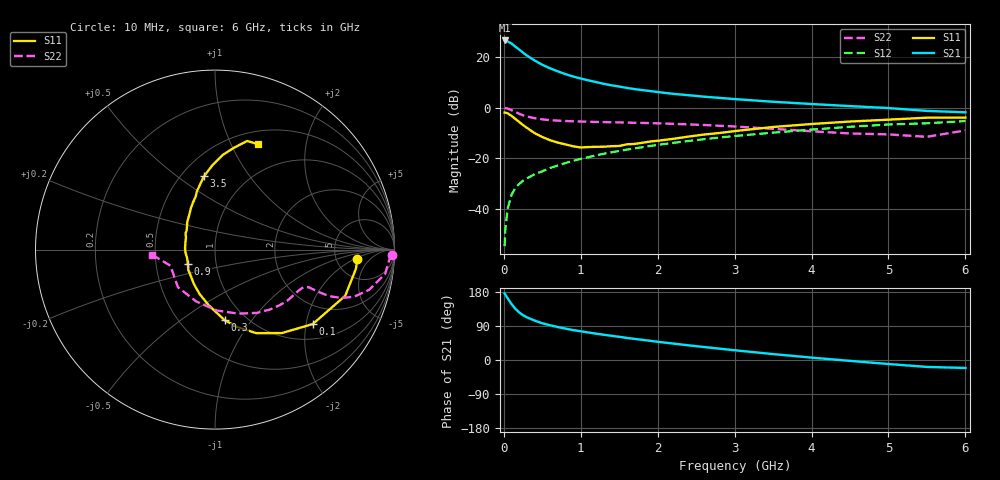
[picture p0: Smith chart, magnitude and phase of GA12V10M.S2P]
! Infineon Technologies  Discrete & RF Semiconductors
! BF775
! Si NPN RF Bipolar Junction Transistor in SOT23
! VCE = 12 V  IC = 10 mA
! Common Emitter S-Parameters:  May  1996
# GHz  S  MA  R  50
!  f  S11  S21  S12  S22
! GHz  MAG  ANG  MAG  ANG  MAG  ANG  MAG  ANG
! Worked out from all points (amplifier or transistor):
!   36 points, 10 MHz to 6 GHz, reference 50 ohm
!   highest |S21| = 26.6 dB at 10 MHz (marker M1)
!   |S21| within 3 dB of that: start of sweep to 173.5 MHz
!   unconditionally stable (mu >= 1): 658.7 MHz to 2.732 GHz
!   at 250 MHz: K = 0.64, MSG = 25.3 dB, |S12| = -28.9 dB
!   at 1.4 GHz: K = 1.09, MAG = 11.4 dB, |S12| = -17.7 dB
!   at 6 GHz: K = 0.87, MSG = 1.7 dB, |S12| = -5.3 dB
!   S11 on the Smith chart (normalised r, x): 10 MHz: 8.07, -2.38; 100 MHz: 1.40, -2.19; 300 MHz: 0.80, -0.75; 900 MHz: 0.73, -0.12; 3.5 GHz: 0.64, +0.63; 6 GHz: 0.65, +1.28
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0.01  0.7955 -3.9  21.35 175.6  0.0018 84.3  0.986 -1.6
0.02  0.7924 -7.7  20.83 172.2  0.004 85.1  0.9729 -3.3
0.05  0.7701 -19.5  20.4 162.6  0.01 79.0  0.9577 -8.1
0.1  0.6845 -37.3  18.56 147.7  0.0188 72.0  0.8876 -14.6
0.15  0.5958 -51.3  16.08 135.1  0.0258 66.7  0.8187 -18.7
0.2  0.5188 -63.8  14.09 125.6  0.0307 64.7  0.7551 -20.9
0.25  0.4501 -73.7  12.24 118.0  0.0358 63.2  0.7019 -21.9
0.3  0.3972 -82.2  10.71 112.6  0.0397 63.3  0.6655 -22.2
0.4  0.3117 -96.5  8.562 104.1  0.0478 63.4  0.6163 -22.2
0.5  0.2615 -109.3  7.036 96.9  0.0547 64.1  0.5836 -22.0
0.6  0.2261 -121.0  5.997 91.7  0.0635 65.3  0.564 -21.9
0.7  0.2029 -130.6  5.221 87.0  0.0713 65.4  0.5522 -22.2
0.9  0.1712 -152.2  4.127 79.0  0.0882 65.8  0.5353 -23.2
1.1  0.1653 -173.6  3.457 72.6  0.1045 65.9  0.5243 -25.0
1.3  0.1678 170.4  2.952 66.6  0.1217 65.1  0.5158 -27.0
1.6  0.1877 151.1  2.449 58.2  0.1471 63.5  0.5039 -30.8
2.2  0.2401 126.8  1.873 43.4  0.2 59.5  0.4768 -40.2
2.8  0.3133 110.2  1.558 30.0  0.2546 54.2  0.4364 -51.8
3.5  0.4129 98.6  1.304 15.6  0.3189 46.9  0.3794 -70.1
4.5  0.5293 85.3  1.07 -2.3  0.4166 35.2  0.3071 -110.1
5.5  0.6311 73.5  0.859 -18.3  0.4886 20.1  0.2638 -160.1
6  0.6346 67.6  0.806 -21.0  0.5403 15.9  0.3527 -175.5
